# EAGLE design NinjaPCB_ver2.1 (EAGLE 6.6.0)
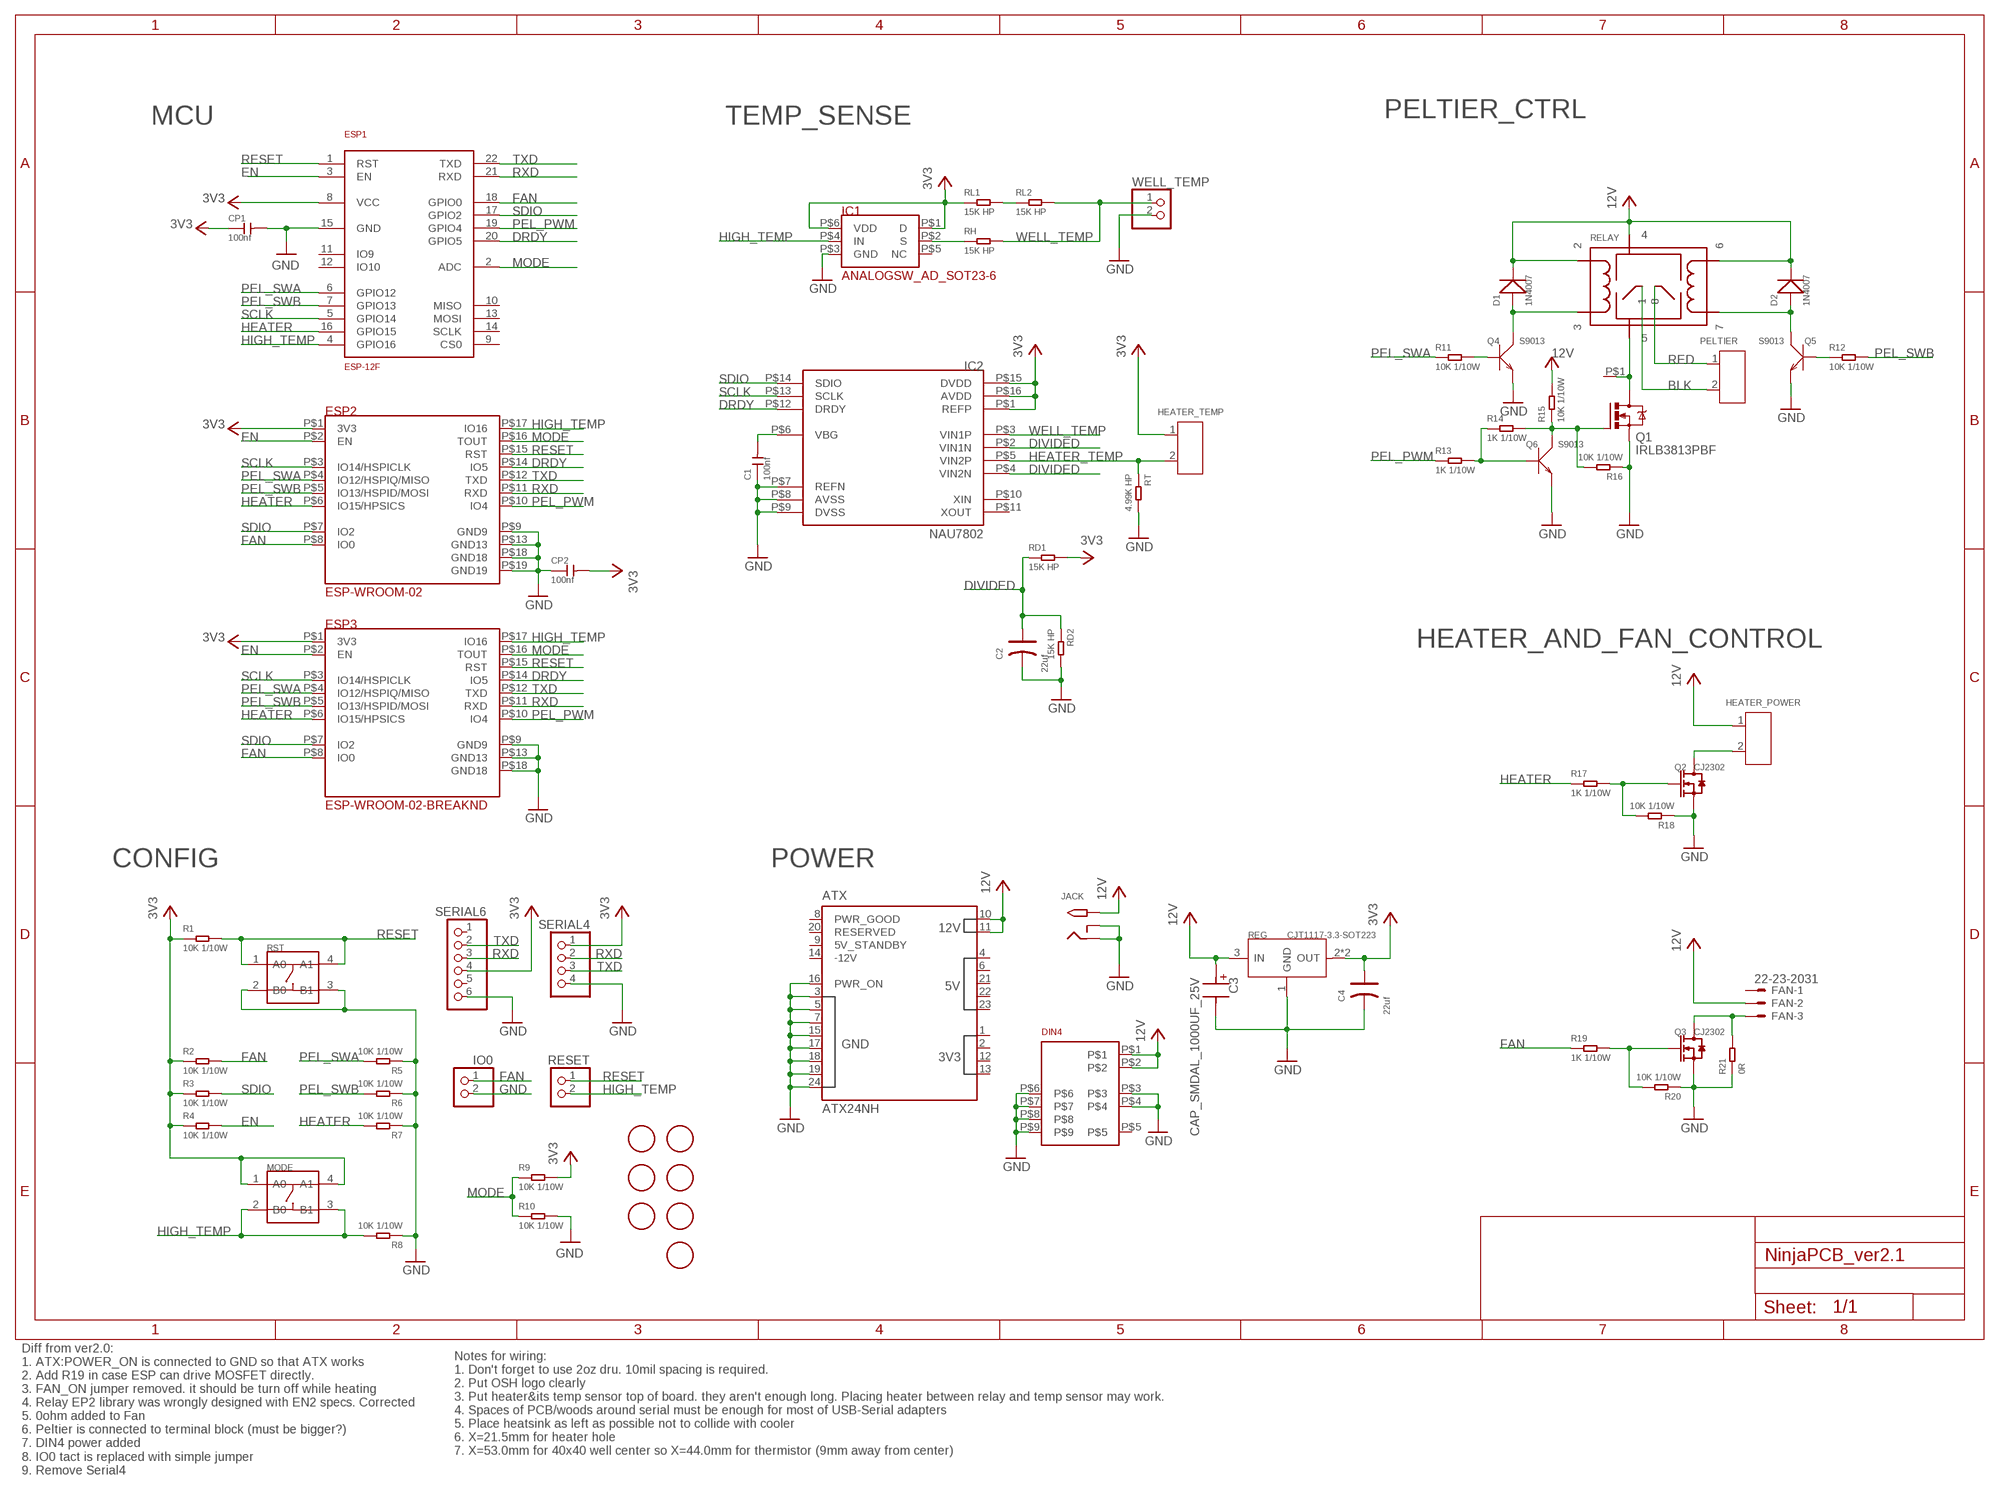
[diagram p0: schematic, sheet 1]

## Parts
ATX  ATX24NH  [ATX24]
C1  100nf  CERAMIC-100NF-50V-10%-X7R(0603)  [C0603]
C2  22uf  TANTALUM-SMD-22UF-16V(AVX-B)  [AVX-B]
C3  CAP_SMDAL_1000UF_25V  [CAP_SMD_AL_D125]
C4  22uf  TANTALUM-SMD-22UF-16V(AVX-B)  [AVX-B]
CP1  100nf  CERAMIC-100NF-50V-10%-X7R(0603)  [C0603]
CP2  100nf  CERAMIC-100NF-50V-10%-X7R(0603)  [C0603]
D1  1N4007  DIODE-GEN-PURPOSE-1KV-1A(DO-214AC)  [DO-214AC]
D2  1N4007  DIODE-GEN-PURPOSE-1KV-1A(DO-214AC)  [DO-214AC]
DIN4  DIN4  [DIN4]
ESP1  ESP-12F  [ESP-12F]
ESP2  ESP-WROOM-02  [ESP-WROOM-02]
ESP3  ESP-WROOM-02-BREAKND  [ESP-WROOM-02-BREAK-NODETAIL]
FAN  22-23-2031  [22-23-2031]
HEATER_POWER  SCREW-TERMINAL-GREEN(2P-3.5)  [H2-3.5-7.0X7.0MM]
HEATER_TEMP  SCREW-TERMINAL-GREEN(2P-3.5)  [H2-3.5-7.0X7.0MM]
HEATSINK  HEAT111PB015  [HEAT11PB015]
IC1  ANALOGSW_AD_SOT23-6  [SOT-23-6]
IC2  NAU7802  [SOP-16]
IO0  PINHD-1X2  [1X02]
JACK  2.1MMJACKTHM-NOOUT  [PJ-102A-NOOUT]
MODE  DIP-SWITCH-TACTILE-SPST-NO/TS-1109(4P-D6.0MM)'TS-1109'  [SW4-6.0X6.0X5.0MM]
PELTIER  SCREW-TERMINAL-GREEN(2P-3.5)  [H2-3.5-7.0X7.0MM]
Q1  IRLB3813PBF  IRF520  [TO220BV]
Q2  CJ2302  SMD-MOSFET-N-CH-20V-2.1A-CJ2302(SOT-23)  [SOT-23]
Q3  CJ2302  SMD-MOSFET-N-CH-20V-2.1A-CJ2302(SOT-23)  [SOT-23]
Q4  S9013  SMD-TRANSISTORS-NPN-25V-500MA-S9013(SOT-23)  [SOT-23]
Q5  S9013  SMD-TRANSISTORS-NPN-25V-500MA-S9013(SOT-23)  [SOT-23]
Q6  S9013  SMD-TRANSISTORS-NPN-25V-500MA-S9013(SOT-23)  [SOT-23]
R1  10K 1/10W  SMD-RES-10K-5%-1/10W(0603)  [R0603]
R2  10K 1/10W  SMD-RES-10K-5%-1/10W(0603)  [R0603]
R3  10K 1/10W  SMD-RES-10K-5%-1/10W(0603)  [R0603]
R4  10K 1/10W  SMD-RES-10K-5%-1/10W(0603)  [R0603]
R5  10K 1/10W  SMD-RES-10K-5%-1/10W(0603)  [R0603]
R6  10K 1/10W  SMD-RES-10K-5%-1/10W(0603)  [R0603]
R7  10K 1/10W  SMD-RES-10K-5%-1/10W(0603)  [R0603]
R8  10K 1/10W  SMD-RES-10K-5%-1/10W(0603)  [R0603]
R9  10K 1/10W  SMD-RES-10K-5%-1/10W(0603)  [R0603]
R10  10K 1/10W  SMD-RES-10K-5%-1/10W(0603)  [R0603]
R11  10K 1/10W  SMD-RES-10K-5%-1/10W(0603)  [R0603]
R12  10K 1/10W  SMD-RES-10K-5%-1/10W(0603)  [R0603]
R13  1K 1/10W  SMD-RES-1K-5%-1/10W(0603)  [R0603]
R14  1K 1/10W  SMD-RES-1K-5%-1/10W(0603)  [R0603]
R15  10K 1/10W  SMD-RES-10K-5%-1/10W(0603)  [R0603]
R16  10K 1/10W  SMD-RES-10K-5%-1/10W(0603)  [R0603]
R17  1K 1/10W  SMD-RES-1K-5%-1/10W(0603)  [R0603]
R18  10K 1/10W  SMD-RES-10K-5%-1/10W(0603)  [R0603]
R19  1K 1/10W  SMD-RES-1K-5%-1/10W(0603)  [R0603]
R20  10K 1/10W  SMD-RES-10K-5%-1/10W(0603)  [R0603]
R21  0R  SMD-RES-0R-5%-1/10W(0603)  [R0603]
RD1  15K HP  R0603  [R0603]
RD2  15K HP  R0603  [R0603]
REG  CJT1117-3.3-SOT223  PMIC-CJT1117-3.3(SOT223)  [SOT-223]
RELAY  NEC-RELAY2EP2  [NEC-EP2]
RESET  PINHD-1X2  [1X02]
RH  15K HP  R0603  [R0603]
RL1  15K HP  R0603  [R0603]
RL2  15K HP  R0603  [R0603]
RST  DIP-SWITCH-TACTILE-SPST-NO/TS-1109(4P-D6.0MM)'TS-1109'  [SW4-6.0X6.0X5.0MM]
RT  4.99K HP  SMD-RES-2K-1%-1/10W(0603)  [R0603]
SERIAL4  PINHD-1X4  [1X04]
SERIAL6  PINHD-1X6  [1X06]
U$3  FIDUCIAL  [FIDUCIAL_1MM]
U$4  FIDUCIAL  [FIDUCIAL_1MM]
U$5  FIDUCIAL  [FIDUCIAL_1MM]
U$7  FIDUCIAL  [FIDUCIAL_1MM]
U$8  FIDUCIAL  [FIDUCIAL_1MM]
U$9  FIDUCIAL  [FIDUCIAL_1MM]
U$10  FIDUCIAL  [FIDUCIAL_1MM]
WELL_TEMP  PINHD-1X2/90  [1X02/90]

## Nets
3V3: C4.+ CP1.1 CP2.2 ESP1.8(VCC) ESP2.P$1(3V3) ESP3.P$1(3V3) HEATER_TEMP.1 IC1.P$1(D) IC1.P$6(VDD) IC2.P$1(REFP) IC2.P$15(DVDD) IC2.P$16(AVDD) MODE.1(A0) MODE.4(A1) R1.1 R2.1 R3.1 R4.1 R9.2 RD1.2 REG.2(OUT) REG.TER(OUT) RL1.1 SERIAL4.1 SERIAL6.4
12V: ATX.10(12V_10) ATX.11(12V_11) C3.P$P D1.2(-) D2.2(-) DIN4.P$1 DIN4.P$2 FAN.2 HEATER_POWER.1 JACK.TIP R15.2 REG.3(IN) RELAY.P$2 RELAY.P$4 RELAY.P$6
BLK: PELTIER.2 RELAY.P$1
DIVIDED: C2.+ IC2.P$2(VIN1N) IC2.P$4(VIN2N) RD1.1 RD2.1
DRDY: ESP1.20(GPIO5) ESP2.P$14(IO5) ESP3.P$14(IO5) IC2.P$12(DRDY)
EN: ESP1.3(EN) ESP2.P$2(EN) ESP3.P$2(EN) R4.2
FAN: ESP1.18(GPIO0) ESP2.P$8(IO0) ESP3.P$8(IO0) IO0.1 R2.2 R19.1
GND: ATX.3(GND3) ATX.5(GND5) ATX.7(GND7) ATX.15(GND15) ATX.16(PWR_ON) ATX.17(GND17) ATX.18(GND18) ATX.19(GND19) ATX.24(GND24) C1.1 C2.- C3.P$M C4.- CP1.2 CP2.1 DIN4.P$3 DIN4.P$4 DIN4.P$6 DIN4.P$7 DIN4.P$8 DIN4.P$9 ESP1.15(GND) ESP2.P$9(GND9) ESP2.P$13(GND13) ESP2.P$18(GND18) ESP2.P$19(GND19) ESP3.P$9(GND9) ESP3.P$13(GND13) ESP3.P$18(GND18) IC1.P$3(GND) IC2.P$7(REFN) IC2.P$8(AVSS) IC2.P$9(DVSS) IO0.2 JACK.RING JACK.RING_SW Q1.S Q2.2(S) Q3.2(S) Q4.2(E) Q5.2(E) Q6.2(E) R5.1 R6.1 R7.1 R8.1 R10.2 R16.1 R18.1 R20.1 R21.1 RD2.2 REG.1(GND) RST.2(B0) RST.3(B1) RT.2 SERIAL4.4 SERIAL6.6 WELL_TEMP.2
HEATER: ESP1.16(GPIO15) ESP2.P$6(IO15/HPSICS) ESP3.P$6(IO15/HPSICS) R7.2 R17.1
HEATER_TEMP: HEATER_TEMP.2 IC2.P$5(VIN2P) RT.1
HIGH_TEMP: ESP1.4(GPIO16) ESP2.P$17(IO16) ESP3.P$17(IO16) IC1.P$4(IN) MODE.2(B0) MODE.3(B1) R8.2 RESET.2
MODE: ESP1.2(ADC) ESP2.P$16(TOUT) ESP3.P$16(TOUT) R9.1 R10.1
N$1: RL1.2 RL2.1
N$2: HEATER_POWER.2 Q2.3(D)
N$3: HEATSINK.P$1 Q1.D RELAY.P$5
N$4: FAN.3 Q3.3(D) R21.2
N$5: Q1.G Q6.3(C) R14.2 R15.1 R16.2
N$8: Q3.1(G) R19.2 R20.2
N$27: IC1.P$2(S) RH.1
N$30: Q6.1(B) R13.2 R14.1
N$32: Q2.1(G) R17.2 R18.2
N$33: D1.1(+) Q4.3(C) RELAY.P$3
N$34: Q4.1(B) R11.2
N$35: Q5.1(B) R12.1
N$36: D2.1(+) Q5.3(C) RELAY.P$7
N$92: C1.2 IC2.P$6(VBG)
PEL_PWM: ESP1.19(GPIO4) ESP2.P$10(IO4) ESP3.P$10(IO4) R13.1
PEL_SWA: ESP1.6(GPIO12) ESP2.P$4(IO12/HSPIQ/MISO) ESP3.P$4(IO12/HSPIQ/MISO) R5.2 R11.1
PEL_SWB: ESP1.7(GPIO13) ESP2.P$5(IO13/HSPID/MOSI) ESP3.P$5(IO13/HSPID/MOSI) R6.2 R12.2
RED: PELTIER.1 RELAY.P$8
RESET: ESP1.1(RST) ESP2.P$15(RST) ESP3.P$15(RST) R1.2 RESET.1 RST.1(A0) RST.4(A1)
RXD: ESP1.21(RXD) ESP2.P$11(RXD) ESP3.P$11(RXD) SERIAL4.2 SERIAL6.3
SCLK: ESP1.5(GPIO14) ESP2.P$3(IO14/HSPICLK) ESP3.P$3(IO14/HSPICLK) IC2.P$13(SCLK)
SDIO: ESP1.17(GPIO2) ESP2.P$7(IO2) ESP3.P$7(IO2) IC2.P$14(SDIO) R3.2
TXD: ESP1.22(TXD) ESP2.P$12(TXD) ESP3.P$12(TXD) SERIAL4.3 SERIAL6.2
WELL_TEMP: IC2.P$3(VIN1P) RH.2 RL2.2 WELL_TEMP.1
Unconnected: ATX.1(3V3_1) ATX.2(3V3_2) ATX.4(5V_4) ATX.6(5V_6) ATX.8(PWR_GOOD) ATX.9(5V_STANDBY) ATX.12(3V3_12) ATX.13(3V3_13) ATX.14(-12V) ATX.20(RESERVED) ATX.21(5V_21) ATX.22(5V_22) ATX.23(5V_23) DIN4.P$5 ESP1.9(CS0) ESP1.10(MISO) ESP1.11(IO9) ESP1.12(IO10) ESP1.13(MOSI) ESP1.14(SCLK) FAN.1 IC1.P$5(NC) IC2.P$10(XIN) IC2.P$11(XOUT) SERIAL6.1 SERIAL6.5

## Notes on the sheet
- MCU | TEMP_SENSE | PELTIER_CTRL
- HEATER_AND_FAN_CONTROL
- CONFIG | POWER
- Notes for wiring: 
  1. Don't forget to use 2oz dru. 10mil spacing is required.
  2. Put OSH logo clearly
  3. Put heater&its temp sensor top of board. they aren't enough long. Placing heater between relay and temp sensor may work.
  4. Spaces of PCB/woods around serial must be enough for most of USB-Serial adapters
  5. Place heatsink as left as possible not to collide with cooler
  6. X=21.5mm for heater hole
  7. X=53.0mm for 40x40 well center so X=44.0mm for thermistor (9mm away from center)
- Diff from ver2.0: 
  1. ATX:POWER_ON is connected to GND so that ATX works
  2. Add R19 in case ESP can drive MOSFET directly.
  3. FAN_ON jumper removed. it should be turn off while heating
  4. Relay EP2 library was wrongly designed with EN2 specs. Corrected
  5. 0ohm added to Fan
  6. Peltier is connected to terminal block (must be bigger?)
  7. DIN4 power added
  8. IO0 tact is replaced with simple jumper
  9. Remove Serial4

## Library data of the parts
ATX = PCR-Connector:ATX24
C1 CP1 CP2 = Seeed-Capacitor:CERAMIC-100NF-50V-10%-X7R(0603): 302010138; MPN: CC0603KRX7R9BB104
C2 C4 = Seeed-Capacitor:TANTALUM-SMD-22UF-16V(AVX-B): 302020013; MPN: TAJB226*016#NJ
C3 = Seeed-OPL-2017-01-Capacitor-akita:CAP_SMDAL_1000UF_25V: SMD CAP Aluminum 1000uF-25V;D12.5*H13.5mm SKU: 302030098
D1 D2 = Seeed-Diode:DIODE-GEN-PURPOSE-1KV-1A(DO-214AC): 304010013; MPN: 1N4007
DIN4 = PCR-Connector:DIN4
ESP1 = Seeed-OPL-2017-01-Sensor-camilo:ESP-12F: 317060163
ESP2 = PCR-Module:ESP-WROOM-02
ESP3 = PCR-Module:ESP-WROOM-02-BREAK
FAN = con-molex:22-23-2031: .100" (2.54mm) Center Header - 3 Pin; MF: MOLEX; MPN: 22-23-2031; OC_FARNELL: 1462950; OC_NEWARK: 30C0862
HEATER_POWER HEATER_TEMP PELTIER = Seeed-Connector:SCREW-TERMINAL-GREEN(2P-3.5): 320110028; VALUE: GREEN-2P-3.5
HEATSINK = PCR-Connector:HEAT1
IC1 = PCR-IC:ANALOGSW_AD_SOT23-6
IC2 = PCR-IC:NAU7802
IO0 RESET WELL_TEMP = pinhead:PINHD-1X2: PIN HEADER
JACK = adafruit:2.1MMJACK: 2.1mm x 5.5mm THM DC jack with internal switch. Digikey part #PJ-102A, 4UCON part #05537 2.1mm x 5.5mm SMT DC jack with internal switch. Digikey part #PJ-002A-SMT, 4UCON part #03267 By microbuilder.eu & adafruit.com
MODE RST = Seeed-Switch:DIP-SWITCH-TACTILE-SPST-NO/TS-1109(4P-D6.0MM): 311020024
Q1 = transistor-power:IRF520: HEXFET Power MOSFET
Q2 Q3 = Seeed-Transistor:SMD-MOSFET-N-CH-20V-2.1A-CJ2302(SOT-23): 305030015; MPN: CJ2302
Q4-Q6 = Seeed-Transistor:SMD-TRANSISTORS-NPN-25V-500MA-S9013(SOT-23): 305010018; MPN: S9013
R1-R12 R15 R16 R18 R20 = Seeed-Resistor:SMD-RES-10K-5%-1/10W(0603): 301010293; MPN: RC0603JR-0710KL
R13 R14 R17 R19 = Seeed-Resistor:SMD-RES-1K-5%-1/10W(0603): 301010291; MPN: RC0603JR-071KL
R21 = Seeed-Resistor:SMD-RES-0R-5%-1/10W(0603): 301010292; MPN: RC0603JR-070RL
RD1 RD2 RH RL1 RL2 = PCR-RCL:R
REG = Seeed-IC:PMIC-CJT1117-3.3(SOT223): 310030097; MPN: CJT1117-3.3
RELAY = PCR-Switch:NEC-RELAY2
RT = Seeed-Resistor:SMD-RES-2K-1%-1/10W(0603): 301010221; MPN: RC0603FR-072KL; VALUE: 2K
SERIAL4 = pinhead:PINHD-1X4: PIN HEADER
SERIAL6 = pinhead:PINHD-1X6: PIN HEADER
U$3-U$5 U$7-U$10 = adafruit:FIDUCIAL: For use by pick and place machines to calibrate the vision/machine, 1mm

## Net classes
1 2A: width 0.406 mm
2 8A: width 2.54 mm

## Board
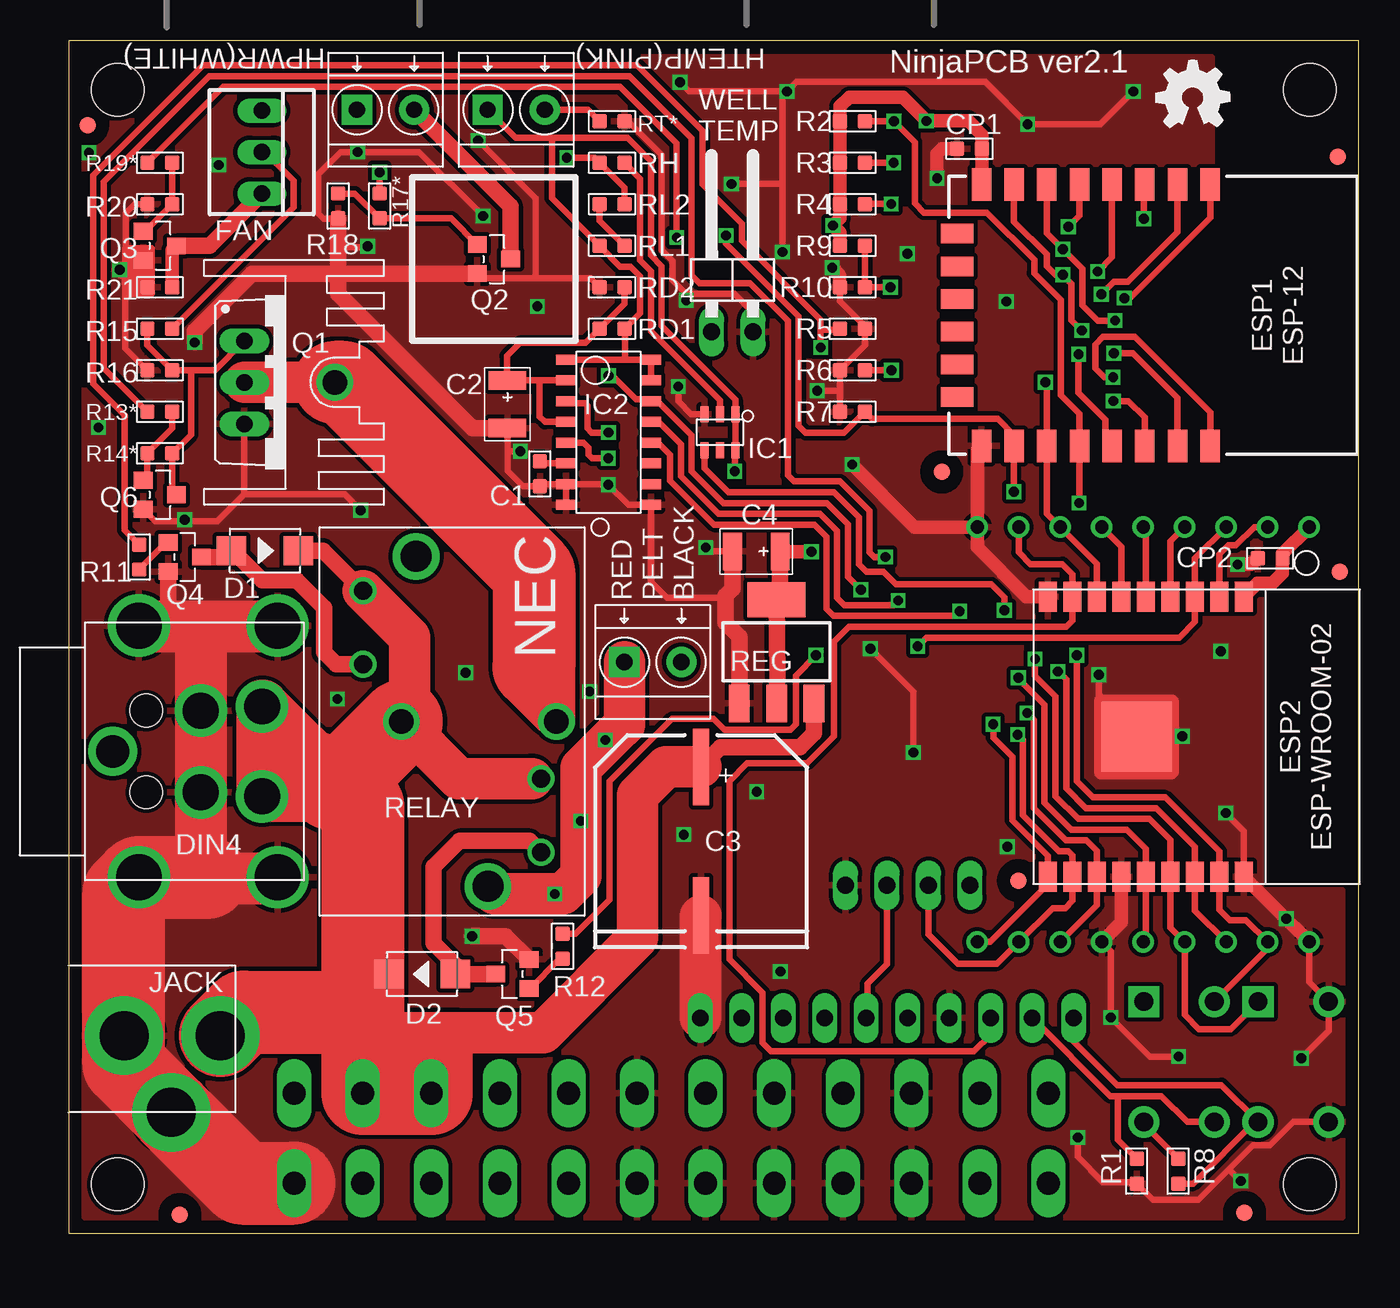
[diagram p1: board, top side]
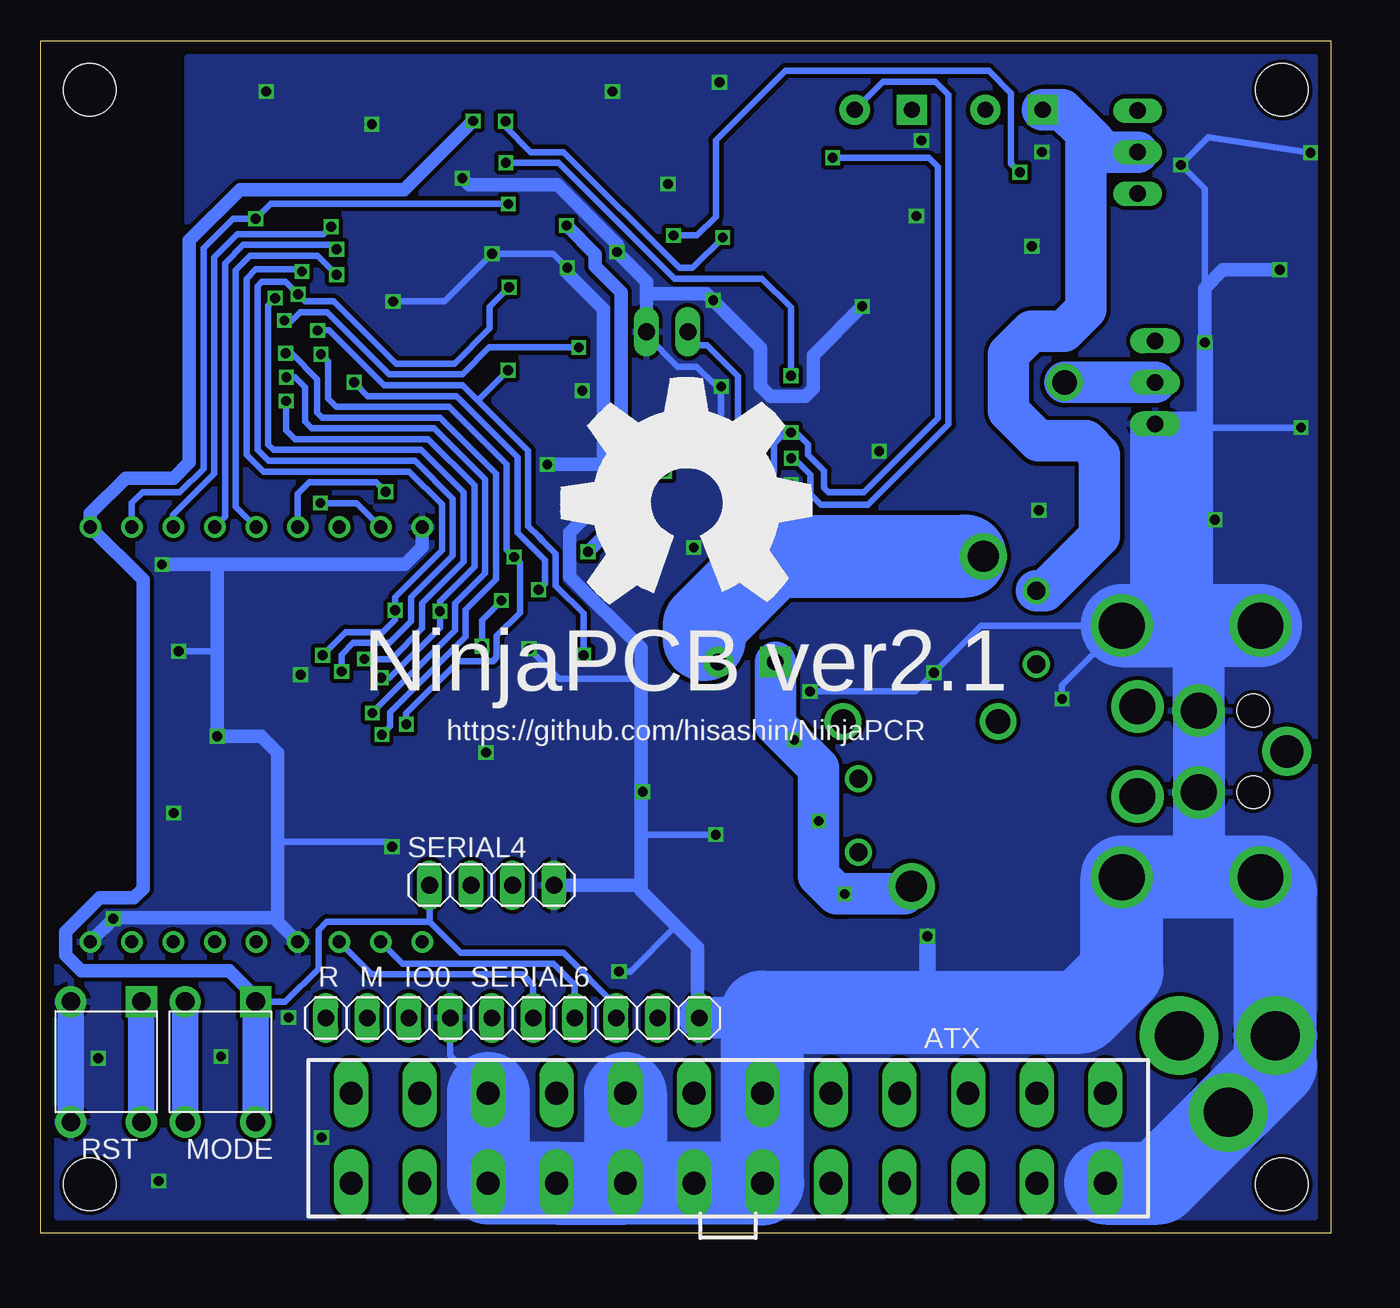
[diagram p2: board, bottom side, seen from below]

Size 79 x 73 mm. Coordinates in mm from the lower left corner, seen from the top.
Outline: 0,0 79,0 79,73 0,73 0,0
Copper layers (1*16): Top 0.035mm / dielectric 1.5mm / Bottom 0.035mm
Design rules "SeeedStudio_2oz": minimum track width 6mil, minimum drill 12mil, track to track 10mil, track to pad 10mil, pad to pad 10mil, via to via 10mil, smd to smd 0mil, copper to edge 10mil, drill to drill 10mil, minimum pad ring 10mil, minimum via ring 6mil, stop-mask expansion 2mil, vias tented up to drill 100mil, thermal gap 10mil
Holes 3.2 mm at 3,3 3,70 76,70 76,3
tKeepout: area 1.4,1.4 to 4.6,4.6; area 74.4,1.4 to 77.6,4.6; area 74.4,68.4 to 77.6,71.6; area 1.4,68.4 to 4.6,71.6

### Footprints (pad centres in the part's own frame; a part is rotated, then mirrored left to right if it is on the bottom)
ATX24 = drill 1.4 long: 1 23.1,-2.75; 2 18.9,-2.75; 3 14.7,-2.75; 4 10.5,-2.75; 5 6.3,-2.75; 6 2.1,-2.75; 7 -2.1,-2.75; 8 -6.3,-2.75; 9 -10.5,-2.75; 10 -14.7,-2.75; 11 -18.9,-2.75; 12 -23.1,-2.75; 13 23.1,2.75; 14 18.9,2.75; 15 14.7,2.75; 16 10.5,2.75; 17 6.3,2.75; 18 2.1,2.75; 19 -2.1,2.75; 20 -6.3,2.75; 21 -10.5,2.75; 22 -14.7,2.75; 23 -18.9,2.75; 24 -23.1,2.75
C0603 = smd 0.889 x 0.889: 1 0,0.762; 2 0,-0.762
AVX-B = smd 1.143 x 2.286: + -1.46,0; - 1.46,0
CAP_SMD_AL_D125 = smd 1 x 4.7: P$M 0,-4.55; P$P 0,4.55
DO-214AC = smd 1.8 x 1.77: 1 -2.042,0; 2 2.042,0
DIN4 = drill 2.2: P$1 -2.75,10.85; P$2 2.75,10.85; P$3 -2.5,7.1; P$4 2.5,7.1 | drill 2: P$5 0,1.7 | drill 2.8: P$6 -7.7,11.8; P$7 -7.7,3.3; P$8 7.7,3.3; P$9 7.7,11.8 | hole 2: -2.5,3.75; 2.5,3.75
ESP-12F = smd 2 x 1.2: 1 -8,3.48; 2 -8,1.48; 3 -8,-0.52; 4 -8,-2.52; 5 -8,-4.52; 6 -8,-6.52; 7 -8,-8.52; 8 -8,-10.52; 15 8,-10.52; 16 8,-8.52; 17 8,-6.52; 18 8,-4.52; 19 8,-2.52; 20 8,-0.52; 21 8,1.48; 22 8,3.48 | smd 1.2 x 2: 9 -5,-12; 10 -3,-12; 11 -1,-12; 12 1,-12; 13 3,-12; 14 5,-12
ESP-WROOM-02 = smd 1.85 x 1.1: P$1 -8.575,12.9; P$2 -8.575,11.4; P$3 -8.575,9.9; P$4 -8.575,8.4; P$5 -8.575,6.9; P$6 -8.575,5.4; P$7 -8.575,3.9; P$8 -8.575,2.4; P$9 -8.575,0.9; P$10 8.575,0.9; P$11 8.575,2.4; P$12 8.575,3.9; P$13 8.575,5.4; P$14 8.575,6.9; P$15 8.575,8.4; P$16 8.575,9.9; P$17 8.575,11.4; P$18 8.575,12.9 | smd 4.3 x 4.3: P$19 0,6.33
ESP-WROOM-02-BREAK-NODETAIL = drill 0.8: P$1 -12.7,10.16; P$2 -12.7,7.62; P$3 -12.7,5.08; P$4 -12.7,2.54; P$5 -12.7,0; P$6 -12.7,-2.54; P$7 -12.7,-5.08; P$8 -12.7,-7.62; P$9 -12.7,-10.16; P$10 12.7,-10.16; P$11 12.7,-7.62; P$12 12.7,-5.08; P$13 12.7,-2.54; P$14 12.7,0; P$15 12.7,2.54; P$16 12.7,5.08; P$17 12.7,7.62; P$18 12.7,10.16
22-23-2031 = drill 1 long: 1 -2.54,0; 2 0,0; 3 2.54,0
H2-3.5-7.0X7.0MM = drill 1 pad 1.85 square: 1 -1.75,0 | drill 1 pad 1.85: 2 1.75,0
HEAT11PB015 = drill 1.5: P$1 0,3
SOT-23-6 = smd 0.5 x 1: P$1 -0.95,-1.1; P$2 0,-1.1; P$3 0.95,-1.1; P$4 0.95,1.1; P$5 0,1.1; P$6 -0.95,1.1
SOP-16 = smd 0.6 x 1.2: P$1 -4.445,-2.6; P$2 -3.175,-2.6; P$3 -1.905,-2.6; P$4 -0.635,-2.6; P$5 0.635,-2.6; P$6 1.905,-2.6; P$7 3.175,-2.6; P$8 4.445,-2.6; P$9 4.445,2.6; P$10 3.175,2.6; P$11 1.905,2.6; P$12 0.635,2.6; P$13 -0.635,2.6; P$14 -1.905,2.6; P$15 -3.175,2.6; P$16 -4.445,2.6
1X02 = drill 1.016 long: 1 -1.27,0; 2 1.27,0
PJ-102A-NOOUT = drill 3 pad 4.8: RING 0.1,-3.39; RING_SW -4.6,-6.29; TIP 0.1,-9.29
SW4-6.0X6.0X5.0MM = drill 1.143 pad 1.905 square: 1 -3.683,2.159 | drill 1.143 pad 1.905: 2 -3.683,-2.159; 3 3.683,-2.159; 4 3.683,2.159
TO220BV = drill 1.016 long: D 0,-2.54; G -2.54,-2.54; S 2.54,-2.54
SOT-23 = smd 1.016 x 1.143: 1 -0.889,-1.016; 2 0.889,-1.016; 3 0,1.016
R0603 = smd 0.889 x 0.889: 1 0,0.762; 2 0,-0.762
SOT-223 = smd 1.27 x 2.286: 1 -2.286,-3.175; 2 0,-3.175; 3 2.286,-3.175 | smd 3.556 x 2.159: TER 0,3.175
NEC-EP2 = drill 1.9: P$1 -10.1,-2.2; P$8 10.1,2.2 | drill 1.1: P$2 -8,-5.45; P$3 -3.5,-5.45; P$6 3.5,5.45; P$7 8,5.45 | drill 1.5: P$4 0,-3.1; P$5 0,6.4
1X04 = drill 1.016 long: 1 -3.81,0; 2 -1.27,0; 3 1.27,0; 4 3.81,0
1X06 = drill 1.016 long: 1 -6.35,0; 2 -3.81,0; 3 -1.27,0; 4 1.27,0; 5 3.81,0; 6 6.35,0
FIDUCIAL_1MM = smd 1 x 1: 1 0,0
1X02/90 = drill 1.016 long: 1 -1.27,-3.81; 2 1.27,-3.81

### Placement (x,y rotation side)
ATX  36.91,5.82 180 bottom
C1  28.86,46.49 180 top
C2  26.87,50.75 270 top
C3  38.73,24 0 top
C4  42.11,41.74 180 top
CP1  55.16,66.4 270 top
CP2  73.57,41.32 90 top
D1  12.02,41.79 0 top
D2  21.64,15.88 180 top
DIN4  1,29.5 270 top
ESP1  66.42,56.2 270 top
ESP2  59.08,30.4 270 top
ESP3  65.8,30.54 270 top
FAN  11.83,66.19 270 top
HEATER_POWER  19.41,68.78 0 top
HEATER_TEMP  27.41,68.78 0 top
HEATSINK  13.3,52.09 270 top
IC1  39.88,49.04 180 top
IC2  33.06,49.04 270 top
IO0  55.19,13.18 0 bottom
JACK  0,12 90 top
MODE  68,10.5 270 bottom
PELTIER  35.77,34.97 0 top
Q1  13.3,52.09 270 top
Q2  26.04,59.63 270 top
Q3  5.59,60.45 270 top
Q4  7.11,41.4 270 top
Q5  27.18,15.88 90 top
Q6  5.59,45.21 270 top
R1  67.94,3.81 0 top
R2  48.01,68.07 90 top
R3  48.01,65.53 90 top
R4  48.01,62.99 90 top
R5  48.01,55.37 270 top
R6  48.01,52.83 90 top
R7  48.01,50.29 90 top
R8  65.41,3.81 180 top
R9  48.01,60.45 270 top
R10  48.01,57.91 270 top
R11  4.32,41.4 0 top
R12  30.25,17.58 180 top
R13  5.59,50.29 90 top
R14  5.59,47.75 90 top
R15  5.59,55.37 90 top
R16  5.59,52.83 90 top
R17  19.05,62.89 0 top
R18  16.51,62.89 180 top
R19  5.59,65.53 90 top
R20  5.59,62.99 90 top
R21  5.59,57.91 90 top
RD1  33.27,55.37 90 top
RD2  33.27,57.91 270 top
REG  43.36,35.61 0 top
RELAY  23.48,31.34 270 top
RESET  60.27,13.18 0 bottom
RH  33.27,65.53 270 top
RL1  33.27,60.45 90 top
RL2  33.27,62.99 90 top
RST  75,10.5 270 bottom
RT  33.27,68.07 90 top
SERIAL4  51.38,21.31 0 bottom
SERIAL6  45.03,13.18 0 bottom
U$1  [OSHW_5MM]  68.83,69.52 0 top
U$3  77.72,65.91 270 top
U$4  6.81,1.14 0 top
U$5  72.01,1.27 0 top
U$6  [OSHW_16MM]  39.5,44.72 0 bottom
U$7  1.17,67.84 0 top
U$8  58.17,21.59 270 top
U$9  53.47,46.61 270 top
U$10  77.85,40.51 270 top
WELL_TEMP  40.64,59 0 top

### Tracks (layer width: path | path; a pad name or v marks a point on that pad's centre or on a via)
3V3  (via drill 0.6)
  Top 0.406: IC2.P$1 34.09,53.48 | 34.09,53.48 IC2.P$16 IC2.P$15 | 34.09,53.48 34.09,55.32 RD1.2 35,56.34 35,58.6 34.42,59.18 33.78,59.18 RL1.1 29.59,63.37 29.59,67.08 | HEATER_TEMP.1 27.36,67.08 29.59,67.08 | 29.59,67.08 34.21,67.08 35.66,65.63 35.66,59.87 36.32,59.21 36.32,55.55 40.83,51.04 IC1.P$1 IC1.P$6 40.79,47.9 v40.79,46.66 | R1.1 65.84,6.68 MODE.4
  Top 0.813: 43.35,34.1 43.41,34.16 | C4.+ 43.66,41.73 v45.49,41.73 | ESP1.8 55.93,64.2 CP1.1 55.93,67.26 55.09,68.1 v52.53,68.1 51.08,69.55 47.8,69.55 47.24,68.99 R2.1 R3.1 R4.1 47.24,62.13 v46.81,61.7 47.24,61.27 R9.2 | ESP2.P$1 72.8,39.8 73.71,39.8 74.31,40.4 CP2.2 74.34,41.61 ESP3.P$1
  Top 1.016: REG.2 43.41,34.16 REG.TER 43.58,39.01 C4.+
  Bottom 0.406: 45.49,41.83 v45.49,41.73 | MODE.1 64.02,14.18 62,16.2 62,18.57 61.49,19.07 55.19,19.07 | 55.19,19.07 53.29,17.17 46.99,17.17 43.76,13.95 SERIAL6.4 | v40.79,46.66 40.82,46.63 43.46,46.63 | SERIAL4.1 55.19,19.07
  Bottom 0.813: v45.49,41.73 43.46,43.76 43.46,46.63 43.46,57.61 45.06,59.21 45.06,59.94 v46.81,61.7 46.79,61.7 | MODE.1 65.84,14.46 67.46,16.08 76.53,16.08 77.47,17.02 77.47,18.47 75.39,20.55 73.3,20.55 72.75,21.11 72.75,40.02 ESP3.P$1 75.96,44.08 73.81,46.23 70.87,46.23 69.9,47.19 69.9,60.78 66.8,63.88 56.74,63.88 v52.53,68.1
  Bottom 1.626: MODE.4 MODE.1
12V
  Top 0.406: FAN.2 12.05,66.19 13.79,64.44 13.79,62.81 R15.2 | DIN4.P$1 11.86,32.26 | 23.5,8.56 22.22,8.56 ATX.10
  Top 0.508: 16.05,27.23 16.48,27.23 16.71,27.46
  Top 1.016: RELAY.P$2 15.58,41.79 D1.2 | D2.2 19.53,15.74 17.32,13.54 17.5,13.36 17.5,12.9 18.01,12.39 ATX.11 | REG.3 45.65,30.61 44.78,29.74 39.91,29.74 C3.P$P
  Top 1.27: 28.37,27.84 RELAY.P$6
  Top 2.54: RELAY.P$2 20.88,36.49 20.88,32.21 20.38,31.71 RELAY.P$4 23.88,27.84 28.37,27.84 | 23.72,12.29 23.5,12.06 23.5,8.56 | 23.72,12.29 20.4,12.29 | 23.72,12.29 29.06,12.29 34.85,18.09 34.85,26.82 36.58,28.55 C3.P$P
  Top 3.175: 15.36,26.75 DIN4.P$2 DIN4.P$1 | 11.89,32.23 11.86,32.26 11.86,32.31 16.71,27.46 | 13.01,28.73 13.56,28.17 14.15,28.17
  Top 5.08: ATX.10 ATX.11 18.01,26.16 16.71,27.46 | RELAY.P$4 16.27,27.23 16.05,27.23 15.11,28.17 14.15,28.17 | JACK.TIP 10.73,13.54 17.32,13.54 17.45,13.54
  Bottom 2.54: 15.01,67.36 15.01,56.57 16.36,55.22 18.34,55.22 19.74,53.82 19.74,50.34 17.91,48.51 15.01,48.51 14.17,47.68 14.17,42.67 17.51,39.34 RELAY.P$2 | 15.01,67.36 16.43,68.78 HEATER_POWER.1 | 15.01,67.36 13.84,66.19 FAN.2
BLK
  Bottom 0.508: 38.38,36.35 37.52,35.49 PELTIER.2 | 22.4,41.45 22.39,41.44 RELAY.P$1
  Bottom 5.08: 38.38,36.35 38.38,37.24 34.16,41.45 22.4,41.45
DIVIDED
  Top 0.406: IC2.P$2 28.8,52.21 | 28.8,52.21 C2.+ 26.85,52.24 26.85,53.72 27.64,54.51 31.65,54.51 RD1.1 34.04,56.9 RD2.1 | IC2.P$4 29.17,49.67 28.85,49.99 28.85,52.16 28.8,52.21
DRDY  (via drill 0.6)
  Top 0.406: IC2.P$12 36.1,48.4 36.83,47.68 36.83,46.08 39.52,43.38 45.67,43.38 46.41,42.65 46.41,38.23 46.84,37.8 54.28,37.8 v54.56,38.08 | ESP3.P$14 65.98,18.01 ESP2.P$14 65.98,23.53 64.8,24.71 61.42,24.71 59.77,26.36 59.77,32.36 58.17,33.96 v58.17,34.01 | ESP1.20 65.9,49.95 64.9,50.95 v63.98,50.95
  Bottom 0.406: v63.98,50.95 63.98,49.17 63.42,48.62 55.27,48.62 52.45,45.8 52.45,40.79 54.56,38.68 v54.56,38.08 54.56,37.08 57.63,34.01 v58.17,34.01
EN  (via drill 0.6)
  Top 0.406: ESP2.P$2 70.48,41.57 71.02,42.11 71.48,42.11 72.6,43.24 ESP3.P$2 | R4.2 48.79,63.02 v50.37,63.02 | ESP1.3 65.84,64.14 v65.84,62.1
  Bottom 0.406: ESP3.P$2 73.42,44.71 72.77,45.36 70.48,45.36 69.04,46.81 69.04,60.3 67.23,62.1 v65.84,62.1 64.92,63.02 v50.37,63.02
FAN  (via drill 0.6)
  Top 0.406: R19.1 9.47,70.18 33.78,70.18 37.24,66.73 v37.24,60.96 | ESP3.P$8 58.18,41.69 58.9,40.97 60.86,40.97 61.48,40.35 ESP2.P$8 61.48,37.5 61.11,37.13 47.78,37.13 46.86,36.22 46.86,30.43 45.21,28.78 41.55,28.78 40.46,27.69 40.46,16.76 42.49,14.73 42.49,11.66 43,11.15 55.45,11.15 56.46,12.17 IO0.1 | R2.2 v50.55,68.07 51.82,66.8 51.82,63.04 52.38,62.48 56.24,62.48 59.13,59.59 59.13,58.78 60.76,57.15 60.76,51.31 61.9,50.16 ESP1.18 61.9,44.73 v61.87,44.7
  Bottom 0.406: ESP3.P$8 59.65,44.7 v61.87,44.7 | v37.24,60.96 39.09,59.11 39.9,59.11 46.99,66.19 49,66.19 50.55,67.74 v50.55,68.07
GND  (via drill 0.6)
  Top 0.406: Q6.2 5.31,43.59 7.01,43.59 | 7.01,43.59 9.09,43.59 10.76,45.26 | 10.76,45.26 Q1.S | 4.83,59.31 Q3.2 | R20.1 4.04,62.99 3.5,62.46 3.5,60.33 | 4.29,59.56 Q3.2 | 3.5,60.33 4.06,59.77 4.37,59.77 Q3.2 | R21.1 4.8,57.91 4.78,57.89 | 5.08,58.42 5.08,57.53 3.48,57.53 | 3.48,57.53 3.48,60.3 | 3.48,60.3 3.76,60.3 3.76,59.38 3.79,59.38 3.79,60.3 5.08,60.3 5.08,59.74 4.01,59.74 4.01,60.07 4.57,60.07 4.57,60.05 | IC2.P$8 IC2.P$7 | IC2.P$7 28.99,45.86 C1.1 27.83,45.73 26.87,46.69 26.87,47.88 | 26.87,47.88 C2.- | RD2.2 31.95,58.47 28.6,58.47 | 28.6,58.47 25.3,58.47 Q2.2 | IC2.P$7 33,45.86 v33.05,45.82 34.27,44.59 IC2.P$9 35.66,39.9 36.65,38.91 40.11,38.91 40.23,39.04 | IC1.P$3 38.13,50.14 37.34,50.93 v37.34,51.84 | RT.2 34.27,68.07 36.32,66.02 36.32,60.2 36.98,59.54 36.98,58.34 37.82,57.51 38.1,57.51 | 38.1,57.51 40.77,57.51 41.91,56.36 WELL_TEMP.2 | R7.1 47.24,51.69 | 47.24,51.69 R6.1 48.77,54.36 R5.1 48.77,55.52 47.24,57.05 R10.2 | 71.04,3.91 69.19,2.06 66.4,2.06 R8.1 65.33,3.12 63.35,3.12 61.8,4.67 v61.8,5.87 | 71.04,3.91 72.52,5.38 73.56,5.38 74.99,6.82 RST.3 | ESP3.P$18 75.96,15.38 RST.2 77.16,12.39 v75.49,10.72 | 4.32,21.79 5.49,21.79 5.56,21.72 | 63.25,28.19 65.96,28.19 v68.2,30.43 | 3.76,58.75 3.66,58.75 | 3.48,60.3 3.5,60.33 | v18.31,60.43 18.26,60.38 16.51,60.38 | v43.99,69.9 43.71,69.62 43.71,64.24 | 43.71,64.24 v43.71,60.07 | v43.99,69.9 44.58,70.48 56.13,70.48 v58.73,67.89 63.2,67.89 v65.2,69.9 | v70.87,25.73 71.98,24.62 ESP2.P$18 | v63.09,34.19 63.09,32.31 64.19,31.22 64.59,31.22 ESP2.P$19 | v71.78,3.2 71.75,3.2 71.04,3.91 | v51.74,29.44 51.74,33.15 v49.1,35.79 | v17.88,44.27 16.9,45.26 10.76,45.26
  Top 0.406: ESP3.P$13 63.83,17.27 v63.83,13.21 66.22,10.82 v67.97,10.82 | v40.59,64.24 43.71,64.24 | v45.85,51.59 47.14,51.59 47.24,51.69 | v74.57,19.25 74.55,19.25 74.05,19.75 | v37.82,57.12 37.82,57.23 38.1,57.51 | R18.1 16.48,62.1 15.62,62.1 15.29,62.43 15.29,64.82 16.66,66.19 v17.7,66.19 21.46,66.19 v25.38,62.28 | v25.07,66.9 28.6,63.37 28.6,58.47 | v27.66,47.88 26.87,47.88 | v39.01,41.99 39.26,41.74 C4.- | 7.01,43.59 v7.11,43.69 | v43.99,69.9 38,69.9 v37.44,70.46 | R16.1 3.48,54.18 3.48,57.53
  Top 0.813: 4.78,57.89 3.96,57.89 3.66,58.19 3.66,58.75 4.19,58.22 4.88,58.22 4.67,58.42 4.67,59.08 4.88,58.88 | 4.88,58.88 4.88,58.29 | 4.88,58.88 4.88,59.82 | ESP2.P$9 58.66,38.98 55.64,41.99 ESP3.P$9 | CP2.1 72.43,40.95 v71.58,40.95 | ESP2.P$19 68.17,30.4 v68.2,30.43 | ESP2.P$13 64.48,19.05 ESP3.P$13 | ESP2.P$18 74.05,19.75 ESP3.P$18 | 63.25,32.59 63.27,32.56 67.56,32.56 67.59,32.54 67.59,28.25 67.54,28.19 63.25,28.19 63.22,28.22 63.22,32.59 | CP1.2 53.49,66.39 53.19,66.09 v53.19,64.59 | ESP3.P$9 51.81,43.24 v47.98,47.07 | ESP3.P$9 55.64,47.94 ESP1.15 | R10.2 47.22,57.94 47.22,58.65 v46.76,59.11
  Top 1.016: 4.47,37.13 4.41,37.2 DIN4.P$7 5.51,37.2 6.1,37.78 Q4.2 | v3.12,58.98 3.76,58.75 Q3.2 | Q2.2 16.43,58.75 | 16.43,58.75 11.25,58.75 7.72,55.22 v7.72,54.53 | R18.1 16.51,60.38 16.51,58.82 | 16.51,58.82 16.43,58.75 | C2.- 24.75,49.29 16.51,57.53 16.51,58.82 | v24.71,18.19 26.77,18.19 Q5.2 | REG.1 41.07,36.52 40.23,37.36 40.23,39.04 40.65,39.46 C4.-
  Top 2.54: C3.P$M 38.68,19.41 SERIAL6.6
  Top 3.175: 4.19,21.77 4.24,21.72 5.56,21.72 8.1,21.72 | 12.72,21.72 8.1,21.72 | 8.1,21.72 8.1,37.13 4.47,37.13 4.24,37.13 4.24,37.16 12.85,37.16
  Top 5.08: 4.12,21.61 DIN4.P$8 4.32,21.79 | 4.32,21.79 8.46,21.79 | 4.32,21.79 3.38,20.85 3.38,10.34 6.29,7.43 JACK.RING_SW 10.62,3.07 ATX.24
  Bottom 0.254: 11.02,49.02 12.17,49.02 12.17,49.58 10.76,49.58 | 10.76,49.58 Q1.S | 9.63,49.58 10.76,49.58
  Bottom 0.406: WELL_TEMP.2 41.91,54.97 40.01,53.06 38.84,53.06 37.62,51.84 v37.34,51.84 37.34,46 36.7,45.36 33.5,45.36 v33.05,45.82 | IO0.2 53.92,10.89 ATX.3 | ATX.7 34.8,8.58 34.8,10.24 | 13.79,3.07 ATX.24 | v7.72,54.53 7.72,63.93 v9.2,65.41 7.49,67.11 v1.25,66.14 | v57.43,57.05 54.28,57.05 v51.36,59.97 47.62,59.97 v46.76,59.11 | v70.56,35.64 68.56,35.64 68.2,35.99 | v49.1,35.79 47.27,33.96 42.24,33.96 | v57.48,23.67 57.78,23.98 64.49,23.98 | v1.83,49.33 7.7,49.33 7.8,49.23 | v37.67,24.41 42.24,24.41 | v42.14,27.03 42.14,26.98 42.24,26.87 | v31.9,33.17 25.45,33.17 v24.31,34.31 21.42,37.2 DIN4.P$6 16.46,33.54 v16.46,32.72 | v43.59,16.03 42.9,16.03 40.09,18.83
  Bottom 0.813: v71.58,40.95 68.38,40.95 | 68.38,40.95 56.69,40.95 55.64,41.99 ESP3.P$9 | 68.38,40.95 68.2,40.77 68.2,35.99 v68.2,30.43 65.51,30.43 64.49,29.41 64.49,23.98 64.49,19.07 | ESP3.P$13 64.49,19.07 | 64.49,19.07 64.75,19.33 74.47,19.33 ESP3.P$18 | v53.19,64.59 52.78,64.19 47.35,64.19 43.71,60.55 v43.71,60.07 41.91,58.27 41.91,57.68 | 44.53,46.81 44.53,56.57 46.76,58.8 v46.76,59.11 | 44.53,46.81 44.53,44.98 46.61,42.9 46.61,40.21 42.24,35.84 42.24,33.96 42.24,26.87 42.24,24.41 42.24,21.31 | v47.98,47.07 44.78,47.07 44.53,46.81 | WELL_TEMP.2 41.91,57.68 | 34.8,3.07 ATX.19 35.2,3.47 35.2,12.9 35.46,13.16 38.71,13.16 38.79,13.23 38.79,17.53 40.09,18.83 42.24,20.98 42.24,21.31 | SERIAL4.4 42.24,21.31 | v28.7,56.74 31.7,53.75 31.7,51.74 32.18,51.26 34.31,51.26 34.92,51.87 34.92,54.2 38.23,57.51 41.73,57.51 41.91,57.68 | v7.72,54.53 7.72,57.86 6.6,58.98 v3.12,58.98
  Bottom 1.016: 9.63,49.58 7.72,47.68 | v7.72,54.53 7.72,46.94 8.48,47.7 8.48,49.23 10.44,49.23 Q1.S 10.62,49.7 10.62,49.81 7.8,49.81 7.8,49.23 7.8,48.74 | v24.71,18.19 24.71,13.54
  Bottom 1.626: RST.2 RST.3
  Bottom 2.54: 9.75,47.78 11.02,47.78 11.02,49.02 | SERIAL6.6 34.81,13.18
  Bottom 3.175: DIN4.P$8 8.1,21.8 DIN4.P$4 DIN4.P$3 8.1,37.2 DIN4.P$7
  Bottom 5.08: ATX.17 ATX.18 ATX.19 | 3.39,10.3 JACK.RING 3.39,20.89 DIN4.P$8 DIN4.P$9 12.8,16.05 15.32,13.54 24.71,13.54 34.81,13.54 34.81,13.18 ATX.7 | DIN4.P$7 DIN4.P$6 9.75,37.2 9.75,47.78 | ATX.17 ATX.16 ATX.15 ATX.3 | 13.79,3.07 10.59,3.07 3.43,10.24 | 34.85,3.02 34.8,3.07 34.8,10.24 | ATX.5 ATX.17
  pour Top (isolate 0.254): 1,72 70,72 70,48 73,48 73,21 78,21 78,1 1,1
  pour Bottom (isolate 0.254): 1,72 70,72 70,48 73,48 73,21 78,21 78,1 1,1
HEATER  (via drill 0.6)
  Top 0.406: R17.1 v19.05,64.95 | ESP3.P$6 64.48,42.03 ESP2.P$6 | v57.89,45.39 57.89,48.19 ESP1.16 57.9,48.86 56.9,49.86 49.2,49.86 R7.2 47.47,49 45.14,49 44.7,49.43 44.7,56.13 40.26,60.58 v40.26,61.09
  Bottom 0.406: v19.05,64.95 19.58,65.48 19.58,69.8 20.95,71.17 33.4,71.17 37.67,66.9 37.67,62.23 38.81,61.09 v40.26,61.09 | ESP3.P$6 63.26,45.27 62.56,45.97 58.47,45.97 v57.89,45.39
HEATER_TEMP  (via drill 0.6)
  Top 0.406: 30.48,48.39 IC2.P$5 31.53,48.4 31.85,48.08 31.85,47.65 32.05,47.45 v33.05,47.45 | RT.1 31.8,68.78 HEATER_TEMP.2
  Bottom 0.406: HEATER_TEMP.2 27.43,70.51 24.23,70.51 23.42,69.7 23.42,49.53 28.35,44.6 31.24,44.6 31.88,45.24 31.88,46.43 32.89,47.45 v33.05,47.45
HIGH_TEMP  (via drill 0.6)
  Top 0.406: IC1.P$4 38.93,46.84 40.41,45.36 46.86,45.36 48.39,43.84 48.39,40.97 48.87,40.49 49.89,40.49 50.65,39.73 56.52,39.73 57.3,38.94 v57.3,38.15 | R8.2 64.26,5.71 64.26,8.38 64.29,8.41 | 64.29,8.41 63.78,8.41 RESET.2 | 64.29,8.41 66.9,8.41 68.49,6.82 MODE.3 | MODE.2 73.42,17.45 ESP3.P$17 72.09,19.18 71.09,19.18 70.48,19.8 ESP2.P$17 70.48,23.38 67.16,26.7 62.71,26.7 61.75,27.66 v61.75,35.38 | ESP1.4 63.9,59.76 v63.02,58.88
  Bottom 0.406: v63.02,58.88 63.14,59 65.84,59 66.4,58.45 66.4,47.68 65.35,46.63 56.44,46.63 54.43,44.63 54.43,41.81 57.3,38.94 v57.3,38.15 57.3,37.57 58.06,36.8 60.33,36.8 v61.75,35.38
  Bottom 1.626: MODE.3 MODE.2
MODE  (via drill 0.6)
  Top 0.406: 48.87,60.55 R9.1 R10.1 v50.32,57.91 | ESP1.2 67.9,61.27 64.87,58.24 64.01,58.24 v63.25,57.48 | ESP3.P$16 68.98,19.75 ESP2.P$16 68.98,23.66 66.6,26.04 62.31,26.04 61.09,27.25 61.09,33.93 60.63,34.39 v60.58,34.39
  Bottom 0.406: v50.32,57.91 51.51,56.72 51.51,55.4 53.67,53.24 57.25,53.24 61.06,57.05 62.81,57.05 v63.25,57.48 64.01,58.24 65.48,58.24 65.73,57.99 65.73,47.98 65.05,47.3 56.08,47.3 53.77,44.98 53.77,41.48 56.31,38.94 56.31,37.47 57.63,36.14 59.87,36.14 60.58,35.43 v60.58,34.39
N$1
  Top 0.406: RL1.2 32.51,61.98 RL2.1
N$2
  Top 1.016: HEATER_POWER.2 27.06,62.88 Q2.3
N$3
  Top 0.406: Q1.D
  Top 1.27: 28.5,34.67 30.4,34.67 30.4,31.32 29.13,31.32 27.13,33.33 28.5,33.33 29.64,32.18 29.64,31.58 RELAY.P$5
  Top 2.54: Q1.D 16.18,52.09
  Top 5.08: HEATSINK.P$1 16.84,52.09 28.5,40.44 28.5,34.67
  Bottom 2.54: Q1.D HEATSINK.P$1
N$4
  Top 0.813: R21.2 6.35,60.2 Q3.3
  Top 1.016: FAN.3 8.63,60.45 Q3.3
N$5
  Top 0.406: Q6.3 6.35,45.47 R14.2 7.49,48.9 7.49,52.83 | Q1.G 8.96,52.83 7.49,52.83 | 7.49,52.83 R16.2 4.83,54.36 R15.1
N$8
  Top 0.406: Q3.1 4.7,61.34 R20.2 R19.2
N$27
  Top 0.406: RH.1 35,64.57 35,59.56 35.66,58.9 35.66,55.22 39.88,51 IC1.P$2
N$30
  Top 0.406: Q6.1 4.83,46.35 R14.1 6.35,49.28 R13.2
N$32
  Top 0.406: R18.2 17.53,63.65 R17.2 23.42,62.13 Q2.1
N$33
  Top 1.016: RELAY.P$3 16.37,34.84 15.65,35.56 15.65,38.3 13.97,39.98 11.86,39.98 10.05,41.79 D1.1 9.59,41.4 Q4.3
N$34
  Top 0.406: Q4.1 5.97,42.29 R11.2
N$35
  Top 0.406: Q5.1 28.25,14.99 30.07,16.82 R12.1
N$36
  Top 1.016: D2.1 23.39,16.18 | D2.1 Q5.3 | 23.47,15.88 D2.1 | RELAY.P$7 28.24,24.03 23.95,24.03 22.35,22.43 22.35,17.75 23.68,16.42 D2.1
N$92
  Top 0.406: IC2.P$6 28.98,47.13 C1.2
PEL_PWM  (via drill 0.6)
  Top 0.406: R13.1 2.16,52.96 2.16,64.39 2.69,64.92 2.79,65.02 8.61,70.84 34.34,70.84 38.15,67.03 38.15,58.65 38.63,58.17 41.73,58.17 44.04,55.85 44.04,46.41 44.42,46.02 47.24,46.02 49.05,44.22 49.05,41.71 49.35,41.4 v50.01,41.4 | ESP3.P$10 56.45,17.84 59.98,21.37 ESP2.P$10 59.98,23.11 57.78,25.3 57.78,29.18 56.62,30.35 v56.62,31.17 | ESP1.19 63.9,48.77 63.5,49.17 63.5,49.81 61.85,51.46 v61.85,53.82
  Bottom 0.406: v61.85,53.82 61.42,53.39 61.42,51.1 60.91,50.6 54,50.6 50.47,47.07 50.47,41.86 v50.01,41.4 49.66,41.05 49.66,38 51.08,36.58 51.08,35.26 51.31,35.03 53.42,35.03 56.62,31.83 v56.62,31.17
PEL_SWA  (via drill 0.6)
  Top 0.406: R11.1 3.43,43.05 3.43,50.09 1.5,52.02 1.5,64.77 8.23,71.5 34.8,71.5 38.81,67.49 38.81,64.21 41.22,61.8 41.22,60.76 46.05,55.93 46.05,55.32 | ESP3.P$4 67.48,42.37 ESP2.P$4 | v64.08,55.88 63.02,55.88 62.08,56.82 62.08,59.05 v60.88,60.25 59.9,61.23 ESP1.6 59.9,63.85 | 46.05,55.32 v46.05,54.23 | R5.2 47.19,55.32 46.05,55.32
  Bottom 0.406: ESP3.P$4 67.72,43.87 67.72,59.38 66.6,60.5 61.14,60.5 v60.88,60.25 | v64.08,55.88 63.63,55.88 63.12,56.39 61.47,56.39 57.66,52.58 53.19,52.58 51.54,54.23 v46.05,54.23
PEL_SWB  (via drill 0.6)
  Top 0.406: ESP3.P$5 65.98,43.07 ESP2.P$5 | R6.2 v50.39,52.83 | R12.2 31.04,18.34 33.12,20.42 33.12,27.66 36.96,31.5 39.5,31.5 40.16,30.84 44.2,30.84 44.53,31.17 44.53,34.14 v45.77,35.38 | v62.05,55.27 61.42,55.91 61.42,58.14 v60.88,58.67 60.43,58.67 59.89,59.21 59.89,59.94 57.9,61.94 ESP1.7
  Bottom 0.406: ESP3.P$5 67.06,44.49 67.06,58.95 66.17,59.84 62.05,59.84 v60.88,58.67 | 52.22,50.98 49.15,47.9 49.15,43.28 48.5,42.63 48.26,42.39 47.47,41.6 47.47,39.65 45.77,37.95 v45.77,35.38 | 52.22,50.98 53.16,51.92 57.99,51.92 61.34,55.27 v62.05,55.27 | v50.39,52.83 52.22,51 52.22,50.98
RED  (via drill 0.6)
  Top 0.254: v32.87,30.2 33.1,30.2 33.47,30.57 | v31.37,25.25 31.37,28.19 31.39,28.22
  Top 0.406: RELAY.P$8 25.65,21.21
  Top 2.54: 25.65,21.21 26.09,20.78 v29.77,20.78 30.28,20.78 31.39,21.89 31.39,28.22 31.39,28.5 33.47,30.57 34.04,31.14 34.04,34.98
  Bottom 2.54: 25.65,21.23 26.11,20.78 v29.77,20.78 30.28,20.78 31.39,21.89 31.39,28.5 34.02,31.13 PELTIER.1
RESET  (via drill 0.6)
  Top 0.406: R1.2 68.86,3.05 72.63,6.82 RST.4 70.59,9.07 64.21,9.07 61.54,11.73 RESET.1 | ESP1.1 69.9,62.18 64.97,57.25 v64.64,57.25 | RST.1 71.16,12.5 69.22,12.5 68.34,13.37 ESP3.P$15 67.48,18.71 ESP2.P$15 67.48,24.09 66.19,25.38 61.82,25.38 60.43,26.77 60.43,32.89 59.18,34.14 v59.18,35.15
  Bottom 0.406: v64.64,57.25 65.08,56.82 65.08,48.28 64.75,47.95 55.7,47.95 53.11,45.36 53.11,41.12 55.65,38.58 55.65,37.03 57.53,35.15 v59.18,35.15
  Bottom 1.626: RST.1 RST.4
RXD  (via drill 0.6)
  Top 0.406: ESP1.21 67.9,51.15 65.18,53.87 v64.01,53.87 | v58.12,30.53 58.45,30.2 58.45,25.6 60.66,23.39 61.21,23.39 61.48,23.13 ESP2.P$11 61.48,20.35 61.04,19.91 60.26,19.91 ESP3.P$11 56.85,16.51 54.46,16.51 52.65,18.31 SERIAL4.2
  Bottom 0.406: SERIAL6.3 46.3,15.21 47.6,16.51 56.85,16.51 ESP3.P$11 | v64.01,53.87 63.65,53.87 62.08,52.3 62.08,50.24 61.77,49.94 54.56,49.94 51.13,46.51 51.13,40.03 52.98,38.18 52.98,36.52 57.61,31.9 57.61,31.04 v58.12,30.53
SCLK  (via drill 0.6)
  Top 0.406: IC2.P$13 36.13,49.67 37.49,48.31 37.49,46.35 39.8,44.04 46.02,44.04 47.07,43 47.07,38.91 47.52,38.46 50.52,38.46 v50.8,38.73 | ESP3.P$3 68.98,41.33 ESP2.P$3 68.98,37.43 68.02,36.47 52.53,36.47 v51.99,35.94 | v61.21,61.62 61.9,62.31 ESP1.5
  Bottom 0.406: ESP3.P$3 70.88,44 68.38,46.51 68.38,59.77 66.98,61.16 61.67,61.16 v61.21,61.62 | v51.99,35.94 51.99,37.54 v50.8,38.73
SDIO  (via drill 0.6)
  Top 0.406: ESP2.P$7 62.98,40.99 ESP3.P$7 59.9,44.06 ESP1.17 59.9,52.01 v59.82,52.09 | v33.07,52.5 33.3,52.5 34.75,51.05 35.55,51.05 IC2.P$14 36.08,50.94 38.15,48.87 38.15,46.66 40.11,44.7 46.43,44.7 47.73,43.41 47.73,40.18 v48.51,39.4 | R3.2 v50.52,65.53
  Bottom 0.406: v50.52,65.53 47.3,65.53 40.21,58.45 34.82,58.45 33.07,56.69 v33.07,52.5 | v59.82,52.09 58.98,51.26 53.54,51.26 49.81,47.52 49.81,42.88 48.13,41.2 48.13,39.78 v48.51,39.4
TXD  (via drill 0.6)
  Top 0.406: ESP3.P$12 62.98,20.09 ESP2.P$12 62.98,23.41 62.33,24.05 61.06,24.05 59.11,26.01 59.11,31.45 v58.7,31.85 | ESP1.22 69.9,50.27 65.28,54.89 63.35,54.89 62.87,54.41 62.87,52.96 63.42,52.4 v63.96,52.4 | SERIAL4.3 50.11,16.48 48.91,15.28 48.91,13.25 SERIAL6.2
  Bottom 0.406: SERIAL6.2 48.84,15.21 49.48,15.85 58.73,15.85 ESP3.P$12 | v63.96,52.4 63.42,52.4 62.81,51.79 62.81,49.68 62.41,49.28 54.91,49.28 51.79,46.15 51.79,40.41 53.65,38.56 53.65,36.93 58.7,31.88 v58.7,31.85
WELL_TEMP  (via drill 0.6)
  Top 0.406: RL2.2 34.04,64.01 RH.2 32.21,65.84 v30.5,65.84 | v33.07,49.02 32.03,49.02 31.77,49.28 31.77,50.65 31.62,50.8 30.61,50.8 IC2.P$3
  Bottom 0.406: v30.5,65.84 24.61,65.84 24.08,65.3 24.08,49.89 28.6,45.36 30.76,45.36 31.04,45.64 31.04,46.69 32.03,47.68 32.03,48.31 32.74,49.02 v33.07,49.02 33.43,49.02 34.11,48.34 34.11,46.58 34.52,46.18 36.07,46.18 36.32,46.43 36.32,52.48 38.2,54.36 38.79,54.36 39.37,54.94 WELL_TEMP.1

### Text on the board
tPlace: HPWR(WHITE) | HTEMP(PINK) | NinjaPCB ver2.1 | R2 | RT* | WELL / TEMP | CP1 | R19* | R3 | R17* | RH | R20 | R4 | FAN | RL2 | Q3 | R18 | R9 | RL1 | R10 | R21 | Q2 | RD2 | R15 | R5 | ESP1 / ESP-12 | RD1 | Q1 | R16 | C2 | R6 | R13* | R7 | IC2 | R14* | IC1 | Q6 | C1 | C4 | CP2 | R11 | Q4 | D1 | RED / PELT / BLACK | REG | ESP2 / ESP-WROOM-02 | + | RELAY | DIN4 | C3 | JACK | R12 | D2 | Q5 | R1 | R8
bPlace: NinjaPCB ver2.1 | https://github.com/hisashin/NinjaPCR | SERIAL4 | SERIAL6 | IO0 | M | R | ATX | MODE | RST
tDocu: pipe | lid | well | center | 79 x 73 mm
